(* Logix 5000 AddOnInstructionDefinition export EH_Liquiphant_FTL43_IOL; software revision 38.00 *)

TYPE EH_CommAOI_Data :
STRUCT
   Device_Comm_Error : BOOL;
   CommSuccess : BOOL;
   CommFailed : BOOL;
   CommTimeOut : BOOL;
   StateDone : BOOL;
   NewState : BOOL;
   OldState : SINT;
   PortSize : SINT;
   DevicePort : SINT;
   MaxState : SINT;
   State : SINT;
   VendorID : INT;
   DeviceID : DINT;
   CyclicData : INT[16];
   AcyclicData : DINT[8];
   ReplayIndex : INT;
   AOI_Diagnostic : DINT;
   ConnectionStatus : DINT;
   OutputData : INT[16];
END_STRUCT
END_TYPE

ADD_ON_INSTRUCTION EH_Liquiphant_FTL43_IOL   (* revision 1.2, vendor Endress+Hauser *)
// Liquiphant FTL 43  Rev 1 IO-Link
// Revision note:
// 1.2 Added HeartbeatVerification
// 1.1 Changed the Datatype from Unsigned to Signed
// Add Disconnect check
VAR_IN_OUT
   DataToSend : INT[10]; {required}
   CommAOIBusy : DINT; {required}
   ActiveComPort : DINT; {required}
   DeviceAOISendRequest : DINT; {required}
   CommError : INT; {required}
   DeviceData : EH_CommAOI_Data; {required}
END_VAR
VAR_INPUT
   iSetSimulation : BOOL; {visible}
   iSimulationVariable : INT; {visible}
   iSetSensorFrequency : REAL; {visible}
   iReadStrengthFork : BOOL; {visible}
   iStart_HeartbeatVerification : BOOL; {visible}
END_VAR
VAR_OUTPUT
   qVendor_ID : DINT; {access Read Only, visible}
   qDevice_ID : DINT; {access Read Only, visible}
   qSensorFrequency : REAL; {access None, visible}
   qExtendedDeviceStatus : INT; {access Read Only, visible}
   qSSC1_1 : BOOL; {access Read Only, visible}
   qSSC1_2 : BOOL; {access Read Only, visible}
   qSignalStrengthOfFork : REAL; {access Read Only, visible}
   qVerificationID : DINT; {visible}
   qPassed : BOOL; {access None, visible}
   qFailed : BOOL; {access None, visible}
   qAOI_Diagnostic : DINT; {access Read Only, visible}
END_VAR
VAR_IN_OUT
   qAOI_Diagnostic_String : STRING; {required}
END_VAR
VAR_OUTPUT
   qActual_Diagnostics_Code : DINT; {access Read Only, visible}
END_VAR
VAR_IN_OUT
   qActual_Diagnostics_String : STRING; {required}
END_VAR
VAR_OUTPUT
   qLast_Diagnostics_Code : DINT; {visible}
END_VAR
VAR_IN_OUT
   qLast_Diagnostics_String : STRING; {required}
END_VAR
VAR_OUTPUT
   qCommError : DINT; {access None}
   qCommunicationBusy : DINT; {access Read Only, visible}
   qDeviceConnectionError : BOOL; {access Read Only, visible}
   qFoamIndex : REAL; {access Read Only}
   qFoamDetected : BOOL; {access Read Only}
   qBuildupIndex : REAL; {access Read Only}
   qBuildupDetected : BOOL; {access Read Only}
END_VAR
VAR
   Temp_DINT : DINT; {access None}
   CMD_Index : INT; {access None}
   CMD_Subindex : INT; {access None}
   CMD_ByteLength : INT; {access None}
   oldCondStatus : INT; {access None}
   oldSetSimulation : SINT; {access None}
   SetSimulation : SINT; {access None}
   oldSetUnit : SINT; {access None}
   oldReadStrengthFork : SINT; {access None}
   Trigger : BOOL; {access None}
   CMD_Rd : BOOL; {access None}
   CMD_Wr : BOOL; {access None}
   SimulationDINT : DINT; {access None}
   AOI_Prio : BOOL; {access None}
   StateMin : DINT; {access None}
   firstTimeDone : BOOL; {access None}
   CondStatusChanged : BOOL; {access None}
   Calc_ExtendedDeviceStatus : DINT; {access None}
   Totalizer1_DINT : DINT; {access None}
   SimActive : BOOL; {access None}
   CondStatusActive : BOOL; {access None}
   ActiveAOI : BOOL; {access None}
   Skip : BOOL; {access None}
   SimChanged : BOOL; {access None}
   ReadStrengthFork : SINT; {access None}
   oldStart_HeartbeatVerification : SINT; {access None}
   Start_HeartbeatVerification : SINT; {access None}
   UnitActive : BOOL; {access None}
   UnitChanged : BOOL; {access None}
   DeviceID : DINT; {access None}
   Calc_SensorFrequ : DINT; {access None}
   FALSE : BOOL; {access None}
   TRUE : BOOL := 1; {access None}
   temp_string1 : STRING; {access None}
   temp_string2 : STRING; {access None}
   qFoamIndexDINT : DINT; {access None}
   qFoamDetectedDINT : DINT; {access None}
   qBuildupIndexDINT : DINT; {access None}
   qBuildupDetectedDINT : DINT; {access None}
   qSignalStrengthOfFork_DINT : DINT; {access None}
   ReadStrengthForkChanged : BOOL; {access None}
   ReadStrengthForkActive : BOOL; {access None}
   HeartbeatVerificationActive : BOOL; {access None}
   HeartbeatVerificationChanged : BOOL; {access None}
END_VAR

ROUTINE Logic   (* structured text *)
// Picomag Communication via AL1323
   // =======================================================================
   // Endress+Hauser Digital Solutions
   // ©Copyright (2024) All Rights Reserved
   // =======================================================================
   // Name:                EH_Liquiphant_FTL43_IOL
   // Version:             1.2
   // Datum:               11.2025
   // Library:             01.01.00
   // Engineering:         Studio5000 V38.00.00
   // Author:              EH
   // =======================================================================
   
   qAOI_Diagnostic := DeviceData.AOI_Diagnostic;
   qCommunicationBusy := CommAOIBusy;
   DeviceID := 9559809;
   StateMin := 0;
   DeviceData.MaxState := 98;
   
   if DeviceData.DevicePort = 0 or DeviceData.DeviceID <> DeviceID or DeviceData.ConnectionStatus <> 1 then
   
   	qVendor_ID := DeviceData.VendorID;
   	qDevice_ID := DeviceData.DeviceID;
   	qSensorFrequency	:= 0;
   	qExtendedDeviceStatus	:= 0;
   	qSSC1_1	:= FALSE;
   	qSSC1_2	:= FALSE;
   	qActual_Diagnostics_Code	:= 0;
   	qLast_Diagnostics_Code	:= 0;
   	qLast_Diagnostics_String	:= '';
   	qSignalStrengthOfFork := 0;
   	qPassed := FALSE;
   	qFailed := FALSE;
   	oldCondStatus := 0;
   	CondStatusChanged := FALSE;
   
   	if DeviceData.DevicePort = 0 then
   
   		qActual_Diagnostics_String	:= 'Device Port is Zero';
   		DeviceData.AOI_Diagnostic.1 := TRUE;
   
   	elsif DeviceData.ConnectionStatus <> 1 then
   
   		qActual_Diagnostics_String	:= 'No Device connected';
   		qDeviceConnectionError := TRUE;
   
   	elsif DeviceData.DeviceID <> DeviceID then
   
   		qActual_Diagnostics_String	:= 'Wrong DeviceID';
   		DeviceData.AOI_Diagnostic.2 := TRUE;
   
   	end_if;
   
   else
   
   	if qActual_Diagnostics_Code = 0  then
   
   		qActual_Diagnostics_String	:= '--------';
   
   	end_if;
   
   	if qLast_Diagnostics_Code = 0 then
   
   		qLast_Diagnostics_String	:= '--------';
   
   	end_if;
   
   	DeviceData.AOI_Diagnostic.1 := FALSE;
   	qDeviceConnectionError := FALSE;
   	DeviceData.AOI_Diagnostic.2  := FALSE;
   
   end_if;
   
   // Case device disconnected during communication to avoid blocking the communication
   if (DeviceData.AOI_Diagnostic.0 or qDeviceConnectionError or DeviceData.AOI_Diagnostic.2) and ActiveAOI and ActiveComPort = DeviceData.DevicePort and CommAOIBusy = 1 then
   
   	DeviceData.State := 0;
   	CommAOIBusy := 0;
   	DeviceAOISendRequest.[DeviceData.DevicePort] := 0;
   	ActiveComPort := 0;
   	ActiveAOI := 0;
   	DataToSend[0] := 0;
   	DataToSend[1] := 0;
   	DataToSend[2] := 0;
   	DataToSend[3] := 0;
   	DataToSend[4] := 0;
   	DataToSend[5] := 0;
   	DataToSend[6] := 0;
   	DataToSend[7] := 0;
   	DataToSend[8] := 0;
   	DataToSend[9] := 0;
   	DeviceData.StateDone := FALSE;
   	DeviceData.NewState := FALSE;
   	DeviceData.OldState := 0;
   	ActiveAOI := FALSE;
   
   end_if;
   
   if not DeviceData.AOI_Diagnostic.0
   
   	and not qDeviceConnectionError
   	and not DeviceData.AOI_Diagnostic.2
   	and DeviceData.DevicePort > 0 then
   
   	//*********************************
   	//Vendor ID
   	//*********************************
   
   		qVendor_ID := DeviceData.VendorID;
   
   	//*********************************
   	//Device ID
   	//*********************************
   
   		qDevice_ID := DeviceData.DeviceID;
   
   	//*********************************
   	// FTL43
   	//*********************************
   
   		Calc_SensorFrequ			:= 0;
   		Calc_ExtendedDeviceStatus	:= 2;
   
   	//*********************************
   	//Process Data Level Linearized
   	//*********************************
   
   		Temp_DINT	 := DeviceData.CyclicData[Calc_SensorFrequ+1];
   		Temp_DINT.8	 := DeviceData.CyclicData[Calc_SensorFrequ+1].8;
   		Temp_DINT.9  := DeviceData.CyclicData[Calc_SensorFrequ+1].9;
   		Temp_DINT.10 := DeviceData.CyclicData[Calc_SensorFrequ+1].10;
   		Temp_DINT.11 := DeviceData.CyclicData[Calc_SensorFrequ+1].11;
   		Temp_DINT.12 := DeviceData.CyclicData[Calc_SensorFrequ+1].12;
   		Temp_DINT.13 := DeviceData.CyclicData[Calc_SensorFrequ+1].13;
   		Temp_DINT.14 := DeviceData.CyclicData[Calc_SensorFrequ+1].14;
   		Temp_DINT.15 := DeviceData.CyclicData[Calc_SensorFrequ+1].15;
   		Temp_DINT.16 := DeviceData.CyclicData[Calc_SensorFrequ].0;
   		Temp_DINT.17 := DeviceData.CyclicData[Calc_SensorFrequ].1;
   		Temp_DINT.18 := DeviceData.CyclicData[Calc_SensorFrequ].2;
   		Temp_DINT.19 := DeviceData.CyclicData[Calc_SensorFrequ].3;
   		Temp_DINT.20 := DeviceData.CyclicData[Calc_SensorFrequ].4;
   		Temp_DINT.21 := DeviceData.CyclicData[Calc_SensorFrequ].5;
   		Temp_DINT.22 := DeviceData.CyclicData[Calc_SensorFrequ].6;
   		Temp_DINT.23 := DeviceData.CyclicData[Calc_SensorFrequ].7;
   		Temp_DINT.24 := DeviceData.CyclicData[Calc_SensorFrequ].8;
   		Temp_DINT.25 := DeviceData.CyclicData[Calc_SensorFrequ].9;
   		Temp_DINT.26 := DeviceData.CyclicData[Calc_SensorFrequ].10;
   		Temp_DINT.27 := DeviceData.CyclicData[Calc_SensorFrequ].11;
   		Temp_DINT.28 := DeviceData.CyclicData[Calc_SensorFrequ].12;
   		Temp_DINT.29 := DeviceData.CyclicData[Calc_SensorFrequ].13;
   		Temp_DINT.30 := DeviceData.CyclicData[Calc_SensorFrequ].14;
   		Temp_DINT.31 := DeviceData.CyclicData[Calc_SensorFrequ].15;
   
   		COP(Temp_DINT,qSensorFrequency,1);
   
   	//*********************************
   	// Extended device Status
   	//*********************************
   
   		qExtendedDeviceStatus.0 := DeviceData.CyclicData[Calc_ExtendedDeviceStatus].8;
   		qExtendedDeviceStatus.1 := DeviceData.CyclicData[Calc_ExtendedDeviceStatus].9;
   		qExtendedDeviceStatus.2 := DeviceData.CyclicData[Calc_ExtendedDeviceStatus].10;
   		qExtendedDeviceStatus.3 := DeviceData.CyclicData[Calc_ExtendedDeviceStatus].11;
   		qExtendedDeviceStatus.4 := DeviceData.CyclicData[Calc_ExtendedDeviceStatus].12;
   		qExtendedDeviceStatus.5 := DeviceData.CyclicData[Calc_ExtendedDeviceStatus].13;
   		qExtendedDeviceStatus.6 := DeviceData.CyclicData[Calc_ExtendedDeviceStatus].14;
   		qExtendedDeviceStatus.7 := DeviceData.CyclicData[Calc_ExtendedDeviceStatus].15;
   
   	//*********************************
   	// Process Parameter SSC
   	//*********************************
   
   		qSSC1_1 := DeviceData.CyclicData[Calc_ExtendedDeviceStatus].0;
   		qSSC1_2 := DeviceData.CyclicData[Calc_ExtendedDeviceStatus].1;
   
   	//*********************************
   	// Checking for Changed Status
   	//*********************************
   
   		SetSimulation.0 := iSetSimulation;
   		ReadStrengthFork.0 := iReadStrengthFork;
   		Start_HeartbeatVerification.0 := iStart_HeartbeatVerification;
   
   	if oldCondStatus <> qExtendedDeviceStatus and not CondStatusChanged then
   
   		CondStatusChanged := TRUE;
   		oldCondStatus := qExtendedDeviceStatus;
   
   	end_if;
   
   	if oldSetSimulation <> SetSimulation and not SimChanged then
   
   		if oldSetSimulation < SetSimulation then
   
   			SimChanged := TRUE;
   
   		end_if;
   
   		oldSetSimulation := SetSimulation;
   
   	end_if;
   
   	if oldReadStrengthFork <> ReadStrengthFork and not ReadStrengthForkChanged then
   
   		if oldReadStrengthFork < ReadStrengthFork then
   
   			ReadStrengthForkChanged := TRUE;
   
   		end_if;
   
   		oldReadStrengthFork := ReadStrengthFork;
   
   	end_if;
   
   	if oldStart_HeartbeatVerification <> Start_HeartbeatVerification and not HeartbeatVerificationChanged then
   
   		if oldStart_HeartbeatVerification < Start_HeartbeatVerification then
   
   			HeartbeatVerificationChanged := TRUE;
   
   		end_if;
   
   		oldStart_HeartbeatVerification := Start_HeartbeatVerification;
   
   	end_if;
   
   	if CondStatusChanged
   	and not ActiveAOI
   	and not CondStatusActive
   	and not Skip then
   
   		DeviceAOISendRequest.[DeviceData.DevicePort] := TRUE;
   		CondStatusActive := TRUE;
   		Skip := TRUE;
   
   	elsif SimChanged
   		and not ActiveAOI
   		and not SimActive
   		and not Skip then
   
   		DeviceAOISendRequest.[DeviceData.DevicePort] := TRUE;
   		SimActive := TRUE;
   		Skip := TRUE;
   
   	elsif ReadStrengthForkChanged
   		and not ActiveAOI
   		and not ReadStrengthForkActive
   		and not Skip then
   
   		DeviceAOISendRequest.[DeviceData.DevicePort] := TRUE;
   		ReadStrengthForkActive := TRUE;
   		Skip := TRUE;
   
   	elsif HeartbeatVerificationChanged
   		and not ActiveAOI
   		and not HeartbeatVerificationActive
   		and not Skip then
   
   		DeviceAOISendRequest.[DeviceData.DevicePort] := TRUE;
   		HeartbeatVerificationActive := TRUE;
   		Skip := TRUE;
   
   	end_if;
   
   	if ActiveComPort = DeviceData.DevicePort then
   
   		AOI_Prio := TRUE;
   
   	else
   
   		AOI_Prio := FALSE;
   
   	end_if;
   
   	if (SimActive or ReadStrengthForkActive  or HeartbeatVerificationActive or CondStatusActive) and CommAOIBusy = 1  and DeviceData.State = 0 and AOI_Prio and not ActiveAOI then
   
   		ActiveAOI := TRUE;
   		Skip := FALSE;
   
   	end_if;
   
   	qCommunicationBusy := CommAOIBusy;
   	qAOI_Diagnostic :=DeviceData.AOI_Diagnostic;
   
   	//*********************************
   	// States for Execution
   	//*********************************
   
   	if ActiveAOI or DeviceData.State = DeviceData.MaxState then
   
   	case DeviceData.State of
   
   		//*********************************
   		0: // Idle
   		//*********************************
   
   			// Initializing
   			Trigger := 0;
   			CMD_Index := 0;
   			CMD_Subindex := 0;
   			CMD_Wr := FALSE;
   			CMD_Rd := FALSE;
   		    CMD_ByteLength := 0;
   
   			if DeviceData.DevicePort = ActiveComPort then
   					DeviceData.CommSuccess := FALSE;
   					DeviceData.CommTimeOut := FALSE;
   					DeviceData.NewState := TRUE;
   					DeviceData.StateDone := FALSE;
   				end_if;
   
   			// Wait for trigger
   			if SimActive then
   
   				DeviceData.AOI_Diagnostic := 0;
   				DeviceData.State := 1;
   
   			elsif ReadStrengthForkActive then
   
   				DeviceData.AOI_Diagnostic := 0;
   				DeviceData.State := 12;
   
   			elsif HeartbeatVerificationActive then
   
   				DeviceData.AOI_Diagnostic := 0;
   				DeviceData.State := 80;
   
   			elsif CondStatusChanged then
   
   				DeviceData.State := 90;
   
   			end_if;
   
   	//*********************************
   	1: // Set Simulation Variable
   	//*********************************
   
   			CMD_Index := 1332;
   			CMD_Subindex := 0;
   			CMD_Wr := TRUE;								// Only Read or Write can be active = 1
   			CMD_Rd := FALSE;
   			CMD_ByteLength := 2;
   			DataToSend[6]:= 0;
   			DataToSend[7]:= 0;
   
   			if iSimulationVariable > 0 then
   
   				DataToSend[6].8 := iSimulationVariable.0;
   				DataToSend[6].9 := iSimulationVariable.1;
   				DataToSend[6].10 := iSimulationVariable.2;
   				DataToSend[6].11 := iSimulationVariable.3;
   				DataToSend[6].12 := iSimulationVariable.4;
   				DataToSend[6].13 := iSimulationVariable.5;
   				DataToSend[6].14 := iSimulationVariable.6;
   				DataToSend[6].15 := iSimulationVariable.7;
   
   			else
   				DataToSend[6] := 0;
   				DataToSend[7] := 0;
   			end_if;
   
   			Trigger := TRUE;
   
   			if DeviceData.NewState then
   				DeviceData.StateDone := TRUE;
   			end_if;
   
   			if  DeviceData.CommSuccess and DeviceData.ReplayIndex = CMD_Index then
   
   				Trigger := FALSE;
   				DeviceData.OldState := DeviceData.State;
   				DeviceData.State := DeviceData.State + 1;
   				DeviceData.CommSuccess := FALSE;
   				DeviceData.AcyclicData[0] := 0;
   				DeviceData.NewState := TRUE;
   
   				elsif DeviceData.CommTimeOut then
   
   					temp_string1 := 'Error in step ';
   					Temp_DINT := DeviceData.State;
   					DTOS(Temp_DINT, temp_string2);
   					CONCAT(temp_string1, temp_string2, qAOI_Diagnostic_String);
   
   					DeviceData.OldState := DeviceData.State;
   					DeviceData.State := DeviceData.MaxState;
   					DeviceData.CommTimeOut := FALSE;
   					DeviceData.AcyclicData[0] := 0;
   					DeviceData.NewState := TRUE;
   
   			end_if;
   
   
   		//*********************************
   		2: // Set Simulation Value
   		//*********************************
   
   			CMD_Index := 8738;
   			CMD_Subindex := 0;
   			CMD_Wr := TRUE;								// Only Read or Write can be active = 1
   			CMD_Rd := FALSE;
   			CMD_ByteLength := 4;
   			DataToSend[6]:= 0;
   			DataToSend[7]:= 0;
   
   		 	COP(iSetSensorFrequency,SimulationDINT,1);		// Copy the Bits from the Real in a DINT
   
   			DataToSend[6].0 :=  SimulationDINT.24;
   			DataToSend[6].1 :=  SimulationDINT.25;
   			DataToSend[6].2 :=  SimulationDINT.26;
   			DataToSend[6].3 :=  SimulationDINT.27;
   			DataToSend[6].4 :=  SimulationDINT.28;
   			DataToSend[6].5 :=  SimulationDINT.29;
   			DataToSend[6].6 :=  SimulationDINT.30;
   			DataToSend[6].7 :=  SimulationDINT.31;
   			DataToSend[6].8 :=  SimulationDINT.16;
   			DataToSend[6].9 :=  SimulationDINT.17;
   			DataToSend[6].10 := SimulationDINT.18;
   			DataToSend[6].11 := SimulationDINT.19;
   			DataToSend[6].12 := SimulationDINT.20;
   			DataToSend[6].13 := SimulationDINT.21;
   			DataToSend[6].14 := SimulationDINT.22;
   			DataToSend[6].15 := SimulationDINT.23;
   			DataToSend[7].0  := SimulationDINT.8;
   			DataToSend[7].1  := SimulationDINT.9;
   			DataToSend[7].2  := SimulationDINT.10;
   			DataToSend[7].3  := SimulationDINT.11;
   			DataToSend[7].4  := SimulationDINT.12;
   			DataToSend[7].5  := SimulationDINT.13;
   			DataToSend[7].6  := SimulationDINT.14;
   			DataToSend[7].7  := SimulationDINT.15;
   			DataToSend[7].8  := SimulationDINT.0;
   			DataToSend[7].9  := SimulationDINT.1;
   			DataToSend[7].10 := SimulationDINT.2;
   			DataToSend[7].11 := SimulationDINT.3;
   			DataToSend[7].12 := SimulationDINT.4;
   			DataToSend[7].13 := SimulationDINT.5;
   			DataToSend[7].14 := SimulationDINT.6;
   			DataToSend[7].15 := SimulationDINT.7;
   
   			Trigger := TRUE;
   
   			if DeviceData.NewState then
   				DeviceData.StateDone := TRUE;
   			end_if;
   
   			if  DeviceData.CommSuccess and DeviceData.ReplayIndex = CMD_Index then
   
   				Trigger := FALSE;
   				DeviceData.OldState := DeviceData.State;
   				DeviceData.State := DeviceData.MaxState;
   				DeviceData.CommSuccess := FALSE;
   				DeviceData.AcyclicData[0] := 0;
   				DeviceData.NewState := TRUE;
   
   		 	elsif DeviceData.CommTimeOut then
   
   				temp_string1 := 'Error in step ';
   				Temp_DINT := DeviceData.State;
   				DTOS(Temp_DINT, temp_string2);
   				CONCAT(temp_string1, temp_string2, qAOI_Diagnostic_String);
   
   				DeviceData.OldState := DeviceData.State;
   				DeviceData.State := DeviceData.MaxState;
   				DeviceData.CommTimeOut := FALSE;
   				DeviceData.AcyclicData[0] := 0;
   				DeviceData.NewState := TRUE;
   
   			end_if;
   
   
   		//*********************************
   		12: // Read Signal Strength of Fork
   		//*********************************
   
   			CMD_Index := 4174;
   			CMD_Subindex := 0;
   			CMD_Wr := FALSE;
   			CMD_Rd := TRUE;
   			CMD_ByteLength := 4;
   			Trigger := TRUE;
   
   			if DeviceData.NewState then
   				DeviceData.StateDone := TRUE;
   			end_if;
   
   			if  DeviceData.CommSuccess and DeviceData.ReplayIndex = CMD_Index then
   
   				qSignalStrengthOfFork_DINT	:= DeviceData.AcyclicData[0];
   	 			COP(qSignalStrengthOfFork_DINT, qSignalStrengthOfFork,1);		// Copy the Bits from the Real in a DINT
   
   				Trigger := FALSE;
   				DeviceData.OldState := DeviceData.State;
   				DeviceData.State := DeviceData.MaxState;
   				DeviceData.CommSuccess := FALSE;
   				DeviceData.AcyclicData[0] := 0;
   				DeviceData.NewState := TRUE;
   
   
   			 elsif DeviceData.CommTimeOut then
   
   				temp_string1 := 'Error in step ';
   				Temp_DINT := DeviceData.State;
   				DTOS(Temp_DINT, temp_string2);
   				CONCAT(temp_string1, temp_string2, qAOI_Diagnostic_String);
   
   				DeviceData.OldState := DeviceData.State;
   				DeviceData.State := DeviceData.MaxState;
   				DeviceData.CommTimeOut := FALSE;
   				DeviceData.AcyclicData[0] := 0;
   				DeviceData.NewState := TRUE;
   
   			end_if;
   
   		//*********************************
   		80: // Check Heartbeat Verification activation
   		//*********************************
   			CMD_Index := 12342;
   			CMD_Subindex := 0;
   			CMD_Wr := FALSE;
   			CMD_Rd := TRUE;
   			CMD_ByteLength := 1;
   			Trigger := TRUE;
   			DataToSend[6]:= 0;
   			DataToSend[7]:= 0;
   
   			if DeviceData.NewState then
   
   				DeviceData.StateDone := TRUE;
   
   			end_if;
   
   			if  DeviceData.CommSuccess and DeviceData.ReplayIndex = CMD_Index then
   
   				if DeviceData.AcyclicData[0] = 1 then
   
   					DeviceData.State := DeviceData.State + 1;
   
   				else
   					qAOI_Diagnostic_String := 'Step 80: Software Option not activated ';
   
   					DeviceData.OldState := DeviceData.State;
   					DeviceData.State := DeviceData.MaxState;
   
   				end_if;
   
   				Trigger := FALSE;
   				DeviceData.CommSuccess := FALSE;
   				DeviceData.AcyclicData[0] := 0;
   				DeviceData.NewState := TRUE;
   
   			 elsif DeviceData.CommTimeOut then
   
   				temp_string1 := 'Error in step ';
   				Temp_DINT := DeviceData.State;
   				DTOS(Temp_DINT, temp_string2);
   				CONCAT(temp_string1, temp_string2, qAOI_Diagnostic_String);
   
   				DeviceData.OldState := DeviceData.State;
   				DeviceData.State := DeviceData.MaxState;
   				DeviceData.CommTimeOut := FALSE;
   				DeviceData.AcyclicData[0] := 0;
   				DeviceData.NewState := TRUE;
   
   			end_if;
   
   		//*********************************
   		81: // Check if Verifivation is ongoing
   		//*********************************
   			CMD_Index := 12323;
   			CMD_Subindex := 0;
   			CMD_Wr := FALSE;
   			CMD_Rd := TRUE;
   			CMD_ByteLength := 2;
   			Trigger := TRUE;
   
   			if DeviceData.NewState then
   
   				DeviceData.StateDone := TRUE;
   
   			end_if;
   
   			if  DeviceData.CommSuccess and DeviceData.ReplayIndex = CMD_Index then
   
   				if DeviceData.AcyclicData[0] <> 8 then
   
   					DeviceData.State := DeviceData.State + 1;
   
   				else
   					qAOI_Diagnostic_String := 'Step 81: Heartbeat Verification already in progress ';
   					DeviceData.OldState := DeviceData.State;
   					DeviceData.State := DeviceData.MaxState;
   					DeviceData.CommTimeOut := FALSE;
   
   				end_if;
   
   				Trigger := FALSE;
   				DeviceData.CommSuccess := FALSE;
   				DeviceData.AcyclicData[0] := 0;
   				DeviceData.NewState := TRUE;
   
   			 elsif DeviceData.CommTimeOut then
   
   				temp_string1 := 'Error in step ';
   				Temp_DINT := DeviceData.State;
   				DTOS(Temp_DINT, temp_string2);
   				CONCAT(temp_string1, temp_string2, qAOI_Diagnostic_String);
   
   				DeviceData.OldState := DeviceData.State;
   				DeviceData.State := DeviceData.MaxState;
   				DeviceData.CommTimeOut := FALSE;
   				DeviceData.AcyclicData[0] := 0;
   				DeviceData.NewState := TRUE;
   
   			end_if;
   
   		//*********************************
   		82: // Start Verification
   		//*********************************
   			CMD_Index := 12325;
   			CMD_Subindex := 0;
   			CMD_Wr := TRUE;
   			CMD_Rd := FALSE;
   			CMD_ByteLength := 2;
   			Trigger := TRUE;
   			DataToSend[6] := 0;
   			DataToSend[7] := 0;
   
   			DataToSend[6].8 := TRUE;
   
   			if DeviceData.NewState then
   
   				DeviceData.StateDone := TRUE;
   
   			end_if;
   
   		if DeviceData.CommSuccess and DeviceData.ReplayIndex = CMD_Index then
   
   		    Trigger := FALSE;
   		    DeviceData.CommSuccess := FALSE;
   		    DeviceData.State := DeviceData.State + 3;
   			DeviceData.AcyclicData[0] := 0;
   			DeviceData.NewState := TRUE;
   
   		elsif DeviceData.CommTimeOut then
   
   		    temp_string1 := 'Error in step ';
   		    Temp_DINT := DeviceData.State;
   		    DTOS(Temp_DINT, temp_string2);
   		    CONCAT(temp_string1, temp_string2, qAOI_Diagnostic_String);
   
   		    DeviceData.OldState := DeviceData.State;
   		    DeviceData.State := DeviceData.MaxState;
   		    DeviceData.CommTimeOut := FALSE;
   			DeviceData.AcyclicData[0] := 0;
   			DeviceData.NewState := TRUE;
   
   		end_if;
   
   
   		//*********************************
   		83: // Intermediate state
   		//*********************************
   			CMD_Index := 36;
   			CMD_Subindex := 0;
   			CMD_Wr := FALSE;
   			CMD_Rd := TRUE;
   			CMD_ByteLength := 1;
   			Trigger := TRUE;
   
   			if DeviceData.NewState then
   
   				DeviceData.StateDone := TRUE;
   
   			end_if;
   
   			if DeviceData.CommSuccess and DeviceData.ReplayIndex = CMD_Index then
   
   			    DeviceData.State := DeviceData.State + 2;
   			    Trigger := FALSE;
   			    DeviceData.CommSuccess := FALSE;
   				DeviceData.AcyclicData[0] := 0;
   				DeviceData.NewState := TRUE;
   
   			elsif DeviceData.CommTimeOut then
   
   			    temp_string1 := 'Error in step ';
   			    Temp_DINT := DeviceData.State;
   			    DTOS(Temp_DINT, temp_string2);
   			    CONCAT(temp_string1, temp_string2, qAOI_Diagnostic_String);
   
   			    DeviceData.OldState := DeviceData.State;
   			    DeviceData.State := DeviceData.MaxState;
   			    DeviceData.CommTimeOut := FALSE;
   				DeviceData.AcyclicData[0] := 0;
   				DeviceData.NewState := TRUE;
   
   			end_if;
   
   		//*********************************
   		84: // Read progress
   		//*********************************
   
   		//*********************************
   		85: // Read status
   		//*********************************
   			CMD_Index := 12323;
   			CMD_Subindex := 0;
   			CMD_Wr := FALSE;
   			CMD_Rd := TRUE;
   			CMD_ByteLength := 2;
   			Trigger := TRUE;
   
   			if DeviceData.NewState then
   
   				DeviceData.StateDone := TRUE;
   
   			end_if;
   
   			if DeviceData.CommSuccess and DeviceData.ReplayIndex = CMD_Index then
   
   			    if DeviceData.AcyclicData[0] = 10 then
   
   			        DeviceData.State := DeviceData.State + 1;
   
   			    elsif DeviceData.AcyclicData[0] = 8 then
   
   					DeviceData.State := DeviceData.State - 2;
   
   			    else
   			        qAOI_Diagnostic_String := 'Step 85: Heartbeat Verification not done';
   			        DeviceData.OldState := DeviceData.State;
   			        DeviceData.State := DeviceData.MaxState;
   			        DeviceData.CommTimeOut := FALSE;
   
   			    end_if;
   
   			    Trigger := FALSE;
   			    DeviceData.CommSuccess := FALSE;
   				DeviceData.AcyclicData[0] := 0;
   				DeviceData.NewState := TRUE;
   
   			elsif DeviceData.CommTimeOut then
   
   			    temp_string1 := 'Error in step ';
   			    Temp_DINT := DeviceData.State;
   			    DTOS(Temp_DINT, temp_string2);
   			    CONCAT(temp_string1, temp_string2, qAOI_Diagnostic_String);
   
   			    DeviceData.OldState := DeviceData.State;
   			    DeviceData.State := DeviceData.MaxState;
   			    DeviceData.CommTimeOut := FALSE;
   				DeviceData.AcyclicData[0] := 0;
   				DeviceData.NewState := TRUE;
   
   			end_if;
   
   		//*********************************
   		86: // Read overall result
   		//*********************************
   			CMD_Index := 1396;
   			CMD_Subindex := 0;
   			CMD_Wr := FALSE;
   			CMD_Rd := TRUE;
   			CMD_ByteLength := 2;
   			Trigger := TRUE;
   
   			if DeviceData.NewState then
   
   				DeviceData.StateDone := TRUE;
   
   			end_if;
   
   			if  DeviceData.CommSuccess and DeviceData.ReplayIndex = CMD_Index then
   
   				if DeviceData.AcyclicData[0] = 1 then
   
   					qPassed := TRUE;
   					qFailed := FALSE;
   
   				else
   
   					qPassed := FALSE;
   					qFailed := TRUE;
   
   				end_if;
   
   				Trigger := FALSE;
   				DeviceData.CommSuccess := FALSE;
   				DeviceData.State := DeviceData.State + 1;
   				DeviceData.AcyclicData[0] := 0;
   				DeviceData.NewState := TRUE;
   
   			 elsif DeviceData.CommTimeOut then
   
   				temp_string1 := 'Error in step ';
   				Temp_DINT := DeviceData.State;
   				DTOS(Temp_DINT, temp_string2);
   				CONCAT(temp_string1, temp_string2, qAOI_Diagnostic_String);
   
   				DeviceData.CommTimeOut := FALSE;
   				DeviceData.OldState := DeviceData.State;
   				DeviceData.State := DeviceData.MaxState;
   				DeviceData.AcyclicData[0] := 0;
   				DeviceData.NewState := TRUE;
   
   			end_if;
   
   		//*********************************
   		87: // Read Verification ID
   		//*********************************
   			CMD_Index := 12321;
   			CMD_Subindex := 0;
   			CMD_Wr := FALSE;
   			CMD_Rd := TRUE;
   			CMD_ByteLength := 2;
   			Trigger := TRUE;
   
   			if DeviceData.NewState then
   
   				DeviceData.StateDone := TRUE;
   
   			end_if;
   
   			if  DeviceData.CommSuccess and DeviceData.ReplayIndex = CMD_Index then
   
   				qVerificationID.0	:= DeviceData.AcyclicData[0].0;
   				qVerificationID.1	:= DeviceData.AcyclicData[0].1;
   				qVerificationID.2	:= DeviceData.AcyclicData[0].2;
   				qVerificationID.3	:= DeviceData.AcyclicData[0].3;
   				qVerificationID.4	:= DeviceData.AcyclicData[0].4;
   				qVerificationID.5	:= DeviceData.AcyclicData[0].5;
   				qVerificationID.6	:= DeviceData.AcyclicData[0].6;
   				qVerificationID.7	:= DeviceData.AcyclicData[0].7;
   				qVerificationID.8	:= DeviceData.AcyclicData[0].8;
   				qVerificationID.9	:= DeviceData.AcyclicData[0].9;
   				qVerificationID.10	:= DeviceData.AcyclicData[0].10;
   				qVerificationID.11	:= DeviceData.AcyclicData[0].11;
   				qVerificationID.12	:= DeviceData.AcyclicData[0].12;
   				qVerificationID.13	:= DeviceData.AcyclicData[0].13;
   				qVerificationID.14	:= DeviceData.AcyclicData[0].14;
   				qVerificationID.15	:= DeviceData.AcyclicData[0].15;
   
   				Trigger := FALSE;
   				DeviceData.CommSuccess := FALSE;
   				DeviceData.OldState := DeviceData.State;
   				DeviceData.State := DeviceData.MaxState;
   				DeviceData.NewState := TRUE;
   
   			 elsif DeviceData.CommTimeOut then
   
   				temp_string1 := 'Error in step ';
   				Temp_DINT := DeviceData.State;
   				DTOS(Temp_DINT, temp_string2);
   				CONCAT(temp_string1, temp_string2, qAOI_Diagnostic_String);
   
   				DeviceData.CommTimeOut := FALSE;
   				DeviceData.OldState := DeviceData.State;
   				DeviceData.State := DeviceData.MaxState;
   				DeviceData.NewState := TRUE;
   
   			end_if;
   
   		//*********************************
   		90: // Actual Diagnostic
   		//*********************************
   
   			CMD_Index := 297;
   			CMD_Subindex := 0;
   			CMD_Wr := FALSE;
   			CMD_Rd := TRUE;
   			CMD_ByteLength := 4;
   			Trigger := TRUE;
   
   			if DeviceData.NewState then
   
   				DeviceData.StateDone := TRUE;
   
   			end_if;
   
   			if  DeviceData.CommSuccess and DeviceData.ReplayIndex = CMD_Index then
   
   				qActual_Diagnostics_Code	:= DeviceData.AcyclicData[0];
   
   				case qActual_Diagnostics_Code of
   
     					0:
   			            qActual_Diagnostics_String := '--------';
   			        16777245:
   			            qActual_Diagnostics_String := 'F081 Sensor initialization faulty';
   			        16777250:
   			            qActual_Diagnostics_String := 'F062 Sensor connection faulty';
   			        16777259:
   			            qActual_Diagnostics_String := 'F801 Supply voltage too low';
   			        16777283:
   			            qActual_Diagnostics_String := 'F803 Loop current faulty';
   			        16777312:
   			            qActual_Diagnostics_String := 'F437 Configuration incompatible';
   			        16777314:
   			            qActual_Diagnostics_String := 'F282 Data storage inconsistent';
   			        16777319:
   			            qActual_Diagnostics_String := 'F242 Firmware incompatible';
   			        16777323:
   			            qActual_Diagnostics_String := 'F252 Module incompatible';
   			        16777336:
   			            qActual_Diagnostics_String := 'F270 Main electronics defective';
   			        16777337:
   			            qActual_Diagnostics_String := 'F272 Main electronics faulty';
   			        16777340:
   			            qActual_Diagnostics_String := 'F270 Main electronics defective';
   			        16777341:
   			            qActual_Diagnostics_String := 'F272 Main electronics faulty';
   			        16777343:
   			            qActual_Diagnostics_String := 'F270 Main electronics defective';
   			        16777344:
   			            qActual_Diagnostics_String := 'F270 Main electronics defective';
   			        16777348:
   			            qActual_Diagnostics_String := 'F270 Main electronics defective';
   			        16777351:
   			            qActual_Diagnostics_String := 'F825 Electronics temperature out of range';
   			        16777355:
   			            qActual_Diagnostics_String := 'F410 Data transfer failed';
   			        16777374:
   			            qActual_Diagnostics_String := 'F283 Memory content inconsistent';
   			        16777375:
   			            qActual_Diagnostics_String := 'F270 Main electronics defective';
   			        16777387:
   			            qActual_Diagnostics_String := 'F270 Main electronics defective';
   			        16777389:
   			            qActual_Diagnostics_String := 'F805 Loop current faulty';
   			        16777441:
   			            qActual_Diagnostics_String := 'F283 Memory content inconsistent';
   			        16777445:
   			            qActual_Diagnostics_String := 'F273 Main electronics defective';
   			        16777446:
   			            qActual_Diagnostics_String := 'F388 Electronics and HistoROM defective';
   			        16777816:
   			            qActual_Diagnostics_String := 'F272 Main electronics faulty';
   			        16778157:
   			            qActual_Diagnostics_String := 'F201 Electronics faulty';
   			        16778194:
   			            qActual_Diagnostics_String := 'F826 Sensor temperature out of range';
   			        16778253:
   			            qActual_Diagnostics_String := 'F062 Sensor connection faulty';
   			        16778254:
   			            qActual_Diagnostics_String := 'F062 Sensor connection faulty';
   			        16778255:
   			            qActual_Diagnostics_String := 'F062 Sensor connection faulty';
   			        16778256:
   			            qActual_Diagnostics_String := 'F062 Sensor connection faulty';
   			        16778279:
   			            qActual_Diagnostics_String := 'F806 Current-loop values deviated';
   			        16778295:
   			            qActual_Diagnostics_String := 'F272 Main electronics faulty';
   			        16778436:
   			            qActual_Diagnostics_String := 'F901 Process alert frequency too high';
   			        16778437:
   			            qActual_Diagnostics_String := 'F900 Process alert frequency too low';
   			        16778445:
   			            qActual_Diagnostics_String := 'F842 Process limit';
   			        16778446:
   			            qActual_Diagnostics_String := 'F007 Sensor defective';
   			        16778447:
   			            qActual_Diagnostics_String := 'F049 Sensor corroded';
   			        16778448:
   			            qActual_Diagnostics_String := 'F042 Sensor corroded';
   			        16778449:
   			            qActual_Diagnostics_String := 'F061 Sensor electronics faulty';
   			        16778457:
   			            qActual_Diagnostics_String := 'F061 Sensor electronics faulty';
   			        16778459:
   			            qActual_Diagnostics_String := 'F061 Sensor electronics faulty';
   			        16778490:
   			            qActual_Diagnostics_String := 'F419 Power cycle required';
   			        16778684:
   			            qActual_Diagnostics_String := 'F004 Sensor defective';
   			        16778685:
   			            qActual_Diagnostics_String := 'F004 Sensor defective';
   			        16778686:
   			            qActual_Diagnostics_String := 'F004 Sensor defective';
   			        16778687:
   			            qActual_Diagnostics_String := 'F004 Sensor defective';
   			        16778688:
   			            qActual_Diagnostics_String := 'F004 Sensor defective';
   			        16778689:
   			            qActual_Diagnostics_String := 'F004 Sensor defective';
   			        16778690:
   			            qActual_Diagnostics_String := 'F004 Sensor defective';
   			        16778691:
   			            qActual_Diagnostics_String := 'F004 Sensor defective';
   			        16778692:
   			            qActual_Diagnostics_String := 'F004 Sensor defective';
   			        16778693:
   			            qActual_Diagnostics_String := 'F004 Sensor defective';
   			        16778694:
   			            qActual_Diagnostics_String := 'F004 Sensor defective';
   			        16778695:
   			            qActual_Diagnostics_String := 'F004 Sensor defective';
   			        16778696:
   			            qActual_Diagnostics_String := 'F004 Sensor defective';
   			        16778697:
   			            qActual_Diagnostics_String := 'F004 Sensor defective';
   			        16778698:
   			            qActual_Diagnostics_String := 'F004 Sensor defective';
   			        16778699:
   			            qActual_Diagnostics_String := 'F004 Sensor defective';
   			        16778700:
   			            qActual_Diagnostics_String := 'F004 Sensor defective';
   			        16778701:
   			            qActual_Diagnostics_String := 'F004 Sensor defective';
   			        16778702:
   			            qActual_Diagnostics_String := 'F004 Sensor defective';
   			        16778703:
   			            qActual_Diagnostics_String := 'F004 Sensor defective';
   			        25165853:
   			            qActual_Diagnostics_String := 'F081 Sensor initialization faulty';
   			        25165858:
   			            qActual_Diagnostics_String := 'F062 Sensor connection faulty';
   			        25165867:
   			            qActual_Diagnostics_String := 'F801 Supply voltage too low';
   			        25165891:
   			            qActual_Diagnostics_String := 'F803 Loop current faulty';
   			        25165920:
   			            qActual_Diagnostics_String := 'F437 Configuration incompatible';
   			        25165922:
   			            qActual_Diagnostics_String := 'F282 Data storage inconsistent';
   			        25165927:
   			            qActual_Diagnostics_String := 'F242 Firmware incompatible';
   			        25165931:
   			            qActual_Diagnostics_String := 'F252 Module incompatible';
   			        25165944:
   			            qActual_Diagnostics_String := 'F270 Main electronics defective';
   			        25165945:
   			            qActual_Diagnostics_String := 'F272 Main electronics faulty';
   			        25165948:
   			            qActual_Diagnostics_String := 'F270 Main electronics defective';
   			        25165949:
   			            qActual_Diagnostics_String := 'F272 Main electronics faulty';
   			        25165951:
   			            qActual_Diagnostics_String := 'F270 Main electronics defective';
   			        25165952:
   			            qActual_Diagnostics_String := 'F270 Main electronics defective';
   			        25165956:
   			            qActual_Diagnostics_String := 'F270 Main electronics defective';
   			        25165959:
   			            qActual_Diagnostics_String := 'F825 Electronics temperature out of range';
   			        25165963:
   			            qActual_Diagnostics_String := 'F410 Data transfer failed';
   			        25165982:
   			            qActual_Diagnostics_String := 'F283 Memory content inconsistent';
   			        25165983:
   			            qActual_Diagnostics_String := 'F270 Main electronics defective';
   			        25165995:
   			            qActual_Diagnostics_String := 'F270 Main electronics defective';
   			        25165997:
   			            qActual_Diagnostics_String := 'F805 Loop current faulty';
   			        25166049:
   			            qActual_Diagnostics_String := 'F283 Memory content inconsistent';
   			        25166053:
   			            qActual_Diagnostics_String := 'F273 Main electronics defective';
   			        25166054:
   			            qActual_Diagnostics_String := 'F388 Electronics and HistoROM defective';
   			        25166424:
   			            qActual_Diagnostics_String := 'F272 Main electronics faulty';
   			        25166765:
   			            qActual_Diagnostics_String := 'F201 Electronics faulty';
   			        25166802:
   			            qActual_Diagnostics_String := 'F826 Sensor temperature out of range';
   			        25166861:
   			            qActual_Diagnostics_String := 'F062 Sensor connection faulty';
   			        25166862:
   			            qActual_Diagnostics_String := 'F062 Sensor connection faulty';
   			        25166863:
   			            qActual_Diagnostics_String := 'F062 Sensor connection faulty';
   			        25166864:
   			            qActual_Diagnostics_String := 'F062 Sensor connection faulty';
   			        25166887:
   			            qActual_Diagnostics_String := 'F806 Current-loop values deviated';
   			        25166903:
   			            qActual_Diagnostics_String := 'F272 Main electronics faulty';
   			        25167044:
   			            qActual_Diagnostics_String := 'F901 Process alert frequency too high';
   			        25167045:
   			            qActual_Diagnostics_String := 'F900 Process alert frequency too low';
   			        25167053:
   			            qActual_Diagnostics_String := 'F842 Process limit';
   			        25167054:
   			            qActual_Diagnostics_String := 'F007 Sensor defective';
   			        25167055:
   			            qActual_Diagnostics_String := 'F049 Sensor corroded';
   			        25167056:
   			            qActual_Diagnostics_String := 'F042 Sensor corroded';
   			        25167057:
   			            qActual_Diagnostics_String := 'F061 Sensor electronics faulty';
   			        25167065:
   			            qActual_Diagnostics_String := 'F061 Sensor electronics faulty';
   			        25167067:
   			            qActual_Diagnostics_String := 'F061 Sensor electronics faulty';
   			        25167098:
   			            qActual_Diagnostics_String := 'F419 Power cycle required';
   			        25167292:
   			            qActual_Diagnostics_String := 'F004 Sensor defective';
   			        25167293:
   			            qActual_Diagnostics_String := 'F004 Sensor defective';
   			        25167294:
   			            qActual_Diagnostics_String := 'F004 Sensor defective';
   			        25167295:
   			            qActual_Diagnostics_String := 'F004 Sensor defective';
   			        25167296:
   			            qActual_Diagnostics_String := 'F004 Sensor defective';
   			        25167297:
   			            qActual_Diagnostics_String := 'F004 Sensor defective';
   			        25167298:
   			            qActual_Diagnostics_String := 'F004 Sensor defective';
   			        25167299:
   			            qActual_Diagnostics_String := 'F004 Sensor defective';
   			        25167300:
   			            qActual_Diagnostics_String := 'F004 Sensor defective';
   			        25167301:
   			            qActual_Diagnostics_String := 'F004 Sensor defective';
   			        25167302:
   			            qActual_Diagnostics_String := 'F004 Sensor defective';
   			        25167303:
   			            qActual_Diagnostics_String := 'F004 Sensor defective';
   			        25167304:
   			            qActual_Diagnostics_String := 'F004 Sensor defective';
   			        25167305:
   			            qActual_Diagnostics_String := 'F004 Sensor defective';
   			        25167306:
   			            qActual_Diagnostics_String := 'F004 Sensor defective';
   			        25167307:
   			            qActual_Diagnostics_String := 'F004 Sensor defective';
   			        25167308:
   			            qActual_Diagnostics_String := 'F004 Sensor defective';
   			        25167309:
   			            qActual_Diagnostics_String := 'F004 Sensor defective';
   			        25167310:
   			            qActual_Diagnostics_String := 'F004 Sensor defective';
   			        25167311:
   			            qActual_Diagnostics_String := 'F004 Sensor defective';
   			        33554445:
   			            qActual_Diagnostics_String := 'C485 Process variable simulation active';
   			        33554446:
   			            qActual_Diagnostics_String := 'C491 Current output simulation active';
   			        33554567:
   			            qActual_Diagnostics_String := 'C825 Electronics temperature out of range';
   			        33554575:
   			            qActual_Diagnostics_String := 'C494 Switch output simulation active';
   			        33554576:
   			            qActual_Diagnostics_String := 'C484 Failure mode simulation active';
   			        33554948:
   			            qActual_Diagnostics_String := 'C412 Processing download';
   			        33555410:
   			            qActual_Diagnostics_String := 'C826 Sensor temperature out of range';
   			        33555459:
   			            qActual_Diagnostics_String := 'C490 Output simulation';
   			        33555495:
   			            qActual_Diagnostics_String := 'C806 Current-loop values deviated';
   			        33555652:
   			            qActual_Diagnostics_String := 'C901 Process alert frequency too high';
   			        33555653:
   			            qActual_Diagnostics_String := 'C900 Process alert frequency too low';
   			        33555654:
   			            qActual_Diagnostics_String := 'C485 Process variable simulation active';
   			        33555660:
   			            qActual_Diagnostics_String := 'C485 Process variable simulation active';
   			        33555663:
   			            qActual_Diagnostics_String := 'C049 Sensor corroded';
   			        33555674:
   			            qActual_Diagnostics_String := 'C485 Process variable simulation active';
   			        41943053:
   			            qActual_Diagnostics_String := 'C485 Process variable simulation active';
   			        41943054:
   			            qActual_Diagnostics_String := 'C491 Current output simulation active';
   			        41943175:
   			            qActual_Diagnostics_String := 'C825 Electronics temperature out of range';
   			        41943183:
   			            qActual_Diagnostics_String := 'C494 Switch output simulation active';
   			        41943184:
   			            qActual_Diagnostics_String := 'C484 Failure mode simulation active';
   			        41943556:
   			            qActual_Diagnostics_String := 'C412 Processing download';
   			        41944018:
   			            qActual_Diagnostics_String := 'C826 Sensor temperature out of range';
   			        41944067:
   			            qActual_Diagnostics_String := 'C490 Output simulation';
   			        41944103:
   			            qActual_Diagnostics_String := 'C806 Current-loop values deviated';
   			        41944260:
   			            qActual_Diagnostics_String := 'C901 Process alert frequency too high';
   			        41944261:
   			            qActual_Diagnostics_String := 'C900 Process alert frequency too low';
   			        41944262:
   			            qActual_Diagnostics_String := 'C485 Process variable simulation active';
   			        41944268:
   			            qActual_Diagnostics_String := 'C485 Process variable simulation active';
   			        41944271:
   			            qActual_Diagnostics_String := 'C049 Sensor corroded';
   			        41944282:
   			            qActual_Diagnostics_String := 'C485 Process variable simulation active';
   			        67108868:
   			            qActual_Diagnostics_String := 'M431 Trim required';
   			        67108970:
   			            qActual_Diagnostics_String := 'M438 Dataset different';
   			        67108999:
   			            qActual_Diagnostics_String := 'M825 Electronics temperature out of range';
   			        67109090:
   			            qActual_Diagnostics_String := 'M287 Memory content inconsistent';
   			        67109839:
   			            qActual_Diagnostics_String := 'M538 Configuration Sensor Unit invalid';
   			        67109842:
   			            qActual_Diagnostics_String := 'M826 Sensor temperature out of range';
   			        67109896:
   			            qActual_Diagnostics_String := 'M807 No Baseline due to insuf. volt. at 20 mA';
   			        67109927:
   			            qActual_Diagnostics_String := 'M806 Current-loop values deviated';
   			        67109944:
   			            qActual_Diagnostics_String := 'M287 Memory content inconsistent';
   			        67110084:
   			            qActual_Diagnostics_String := 'M901 Process alert frequency too high';
   			        67110085:
   			            qActual_Diagnostics_String := 'M900 Process alert frequency too low';
   			        67110095:
   			            qActual_Diagnostics_String := 'M049 Sensor corroded';
   			        75497476:
   			            qActual_Diagnostics_String := 'M431 Trim required';
   			        75497578:
   			            qActual_Diagnostics_String := 'M438 Dataset different';
   			        75497607:
   			            qActual_Diagnostics_String := 'M825 Electronics temperature out of range';
   			        75497698:
   			            qActual_Diagnostics_String := 'M287 Memory content inconsistent';
   			        75498447:
   			            qActual_Diagnostics_String := 'M538 Configuration Sensor Unit invalid';
   			        75498450:
   			            qActual_Diagnostics_String := 'M826 Sensor temperature out of range';
   			        75498504:
   			            qActual_Diagnostics_String := 'M807 No Baseline due to insuf. volt. at 20 mA';
   			        75498535:
   			            qActual_Diagnostics_String := 'M806 Current-loop values deviated';
   			        75498552:
   			            qActual_Diagnostics_String := 'M287 Memory content inconsistent';
   			        75498692:
   			            qActual_Diagnostics_String := 'M901 Process alert frequency too high';
   			        75498693:
   			            qActual_Diagnostics_String := 'M900 Process alert frequency too low';
   			        75498703:
   			            qActual_Diagnostics_String := 'M049 Sensor corroded';
   			        134217772:
   			            qActual_Diagnostics_String := 'S802 Supply voltage too high';
   			        134217863:
   			            qActual_Diagnostics_String := 'S825 Electronics temperature out of range';
   			        134217881:
   			            qActual_Diagnostics_String := 'S441 Current output saturated';
   			        134218194:
   			            qActual_Diagnostics_String := 'S946 Vibration detected';
   			        134218639:
   			            qActual_Diagnostics_String := 'S804 Switch output overloaded';
   			        134218706:
   			            qActual_Diagnostics_String := 'S826 Sensor temperature out of range';
   			        134218791:
   			            qActual_Diagnostics_String := 'S806 Current-loop values deviated';
   			        134218948:
   			            qActual_Diagnostics_String := 'S901 Process alert frequency too high';
   			        134218949:
   			            qActual_Diagnostics_String := 'S900 Process alert frequency too low';
   			        134218959:
   			            qActual_Diagnostics_String := 'S049 Sensor corroded';
   			        142606380:
   			            qActual_Diagnostics_String := 'S802 Supply voltage too high';
   			        142606471:
   			            qActual_Diagnostics_String := 'S825 Electronics temperature out of range';
   			        142606489:
   			            qActual_Diagnostics_String := 'S441 Current output saturated';
   			        142606802:
   			            qActual_Diagnostics_String := 'S946 Vibration detected';
   			        142607247:
   			            qActual_Diagnostics_String := 'S804 Switch output overloaded';
   			        142607314:
   			            qActual_Diagnostics_String := 'S826 Sensor temperature out of range';
   			        142607399:
   			            qActual_Diagnostics_String := 'S806 Current-loop values deviated';
   			        142607556:
   			            qActual_Diagnostics_String := 'S901 Process alert frequency too high';
   			        142607557:
   			            qActual_Diagnostics_String := 'S900 Process alert frequency too low';
   			        142607567:
   			            qActual_Diagnostics_String := 'S049 Sensor corroded';
   			        536871047:
   			            qActual_Diagnostics_String := '825 Electronics temperature out of range';
   			        536871262:
   			            qActual_Diagnostics_String := '495 Diagnostic event simulation active';
   			        536871890:
   			            qActual_Diagnostics_String := '826 Sensor temperature out of range';
   			        536871975:
   			            qActual_Diagnostics_String := '806 Current-loop values deviated';
   			        536872132:
   			            qActual_Diagnostics_String := '901 Process alert frequency too high';
   			        536872133:
   			            qActual_Diagnostics_String := '900 Process alert frequency too low';
   			        536872143:
   			            qActual_Diagnostics_String := '049 Sensor corroded';
   			        545259655:
   			            qActual_Diagnostics_String := '825 Electronics temperature out of range';
   			        545259870:
   			            qActual_Diagnostics_String := '495 Diagnostic event simulation active';
   			        545260498:
   			            qActual_Diagnostics_String := '826 Sensor temperature out of range';
   			        545260583:
   			            qActual_Diagnostics_String := '806 Current-loop values deviated';
   			        545260740:
   			            qActual_Diagnostics_String := '901 Process alert frequency too high';
   			        545260741:
   			            qActual_Diagnostics_String := '900 Process alert frequency too low';
   			        545260751:
   			            qActual_Diagnostics_String := '049 Sensor corroded';
   					else
   						qActual_Diagnostics_String := 'Error Code unknown';
   
   				end_case;
   
   				Trigger := FALSE;
   				DeviceData.OldState := DeviceData.State;
   		        DeviceData.State := DeviceData.State+1;
   				DeviceData.CommSuccess := FALSE;
   				DeviceData.AcyclicData[0] := 0;
   				DeviceData.NewState := TRUE;
   
   			 elsif DeviceData.CommTimeOut then
   
   				temp_string1 := 'Error in step ';
   				Temp_DINT := DeviceData.State;
   				DTOS(Temp_DINT, temp_string2);
   				CONCAT(temp_string1, temp_string2, qAOI_Diagnostic_String);
   
   				DeviceData.OldState := DeviceData.State;
   				DeviceData.State := DeviceData.State + 1;
   				DeviceData.CommTimeOut := FALSE;
   				DeviceData.AcyclicData[0] := 0;
   				DeviceData.NewState := TRUE;
   
   		    end_if;
   
   		//*********************************
   	    91: // Last Diagnostic
   	    //*********************************
   
   		    CMD_Index := 298;
   			CMD_Subindex := 0;
   		    CMD_Wr := FALSE;
   			CMD_Rd := TRUE;
   			CMD_ByteLength := 4;
   			Trigger := TRUE;
   
   			if DeviceData.NewState then
   
   				DeviceData.StateDone := TRUE;
   
   			end_if;
   
   			if  DeviceData.CommSuccess and DeviceData.ReplayIndex = CMD_Index then
   
   				qLast_Diagnostics_Code	:= DeviceData.AcyclicData[0];
   
   				case qLast_Diagnostics_Code of
   					0:
   			            qLast_Diagnostics_String := '--------';
   			        16777245:
   			            qLast_Diagnostics_String := 'F081 Sensor initialization faulty';
   			        16777250:
   			            qLast_Diagnostics_String := 'F062 Sensor connection faulty';
   			        16777259:
   			            qLast_Diagnostics_String := 'F801 Supply voltage too low';
   			        16777283:
   			            qLast_Diagnostics_String := 'F803 Loop current faulty';
   			        16777312:
   			            qLast_Diagnostics_String := 'F437 Configuration incompatible';
   			        16777314:
   			            qLast_Diagnostics_String := 'F282 Data storage inconsistent';
   			        16777319:
   			            qLast_Diagnostics_String := 'F242 Firmware incompatible';
   			        16777323:
   			            qLast_Diagnostics_String := 'F252 Module incompatible';
   			        16777336:
   			            qLast_Diagnostics_String := 'F270 Main electronics defective';
   			        16777337:
   			            qLast_Diagnostics_String := 'F272 Main electronics faulty';
   			        16777340:
   			            qLast_Diagnostics_String := 'F270 Main electronics defective';
   			        16777341:
   			            qLast_Diagnostics_String := 'F272 Main electronics faulty';
   			        16777343:
   			            qLast_Diagnostics_String := 'F270 Main electronics defective';
   			        16777344:
   			            qLast_Diagnostics_String := 'F270 Main electronics defective';
   			        16777348:
   			            qLast_Diagnostics_String := 'F270 Main electronics defective';
   			        16777351:
   			            qLast_Diagnostics_String := 'F825 Electronics temperature out of range';
   			        16777355:
   			            qLast_Diagnostics_String := 'F410 Data transfer failed';
   			        16777374:
   			            qLast_Diagnostics_String := 'F283 Memory content inconsistent';
   			        16777375:
   			            qLast_Diagnostics_String := 'F270 Main electronics defective';
   			        16777387:
   			            qLast_Diagnostics_String := 'F270 Main electronics defective';
   			        16777389:
   			            qLast_Diagnostics_String := 'F805 Loop current faulty';
   			        16777441:
   			            qLast_Diagnostics_String := 'F283 Memory content inconsistent';
   			        16777445:
   			            qLast_Diagnostics_String := 'F273 Main electronics defective';
   			        16777446:
   			            qLast_Diagnostics_String := 'F388 Electronics and HistoROM defective';
   			        16777816:
   			            qLast_Diagnostics_String := 'F272 Main electronics faulty';
   			        16778157:
   			            qLast_Diagnostics_String := 'F201 Electronics faulty';
   			        16778194:
   			            qLast_Diagnostics_String := 'F826 Sensor temperature out of range';
   			        16778253:
   			            qLast_Diagnostics_String := 'F062 Sensor connection faulty';
   			        16778254:
   			            qLast_Diagnostics_String := 'F062 Sensor connection faulty';
   			        16778255:
   			            qLast_Diagnostics_String := 'F062 Sensor connection faulty';
   			        16778256:
   			            qLast_Diagnostics_String := 'F062 Sensor connection faulty';
   			        16778279:
   			            qLast_Diagnostics_String := 'F806 Current-loop values deviated';
   			        16778295:
   			            qLast_Diagnostics_String := 'F272 Main electronics faulty';
   			        16778436:
   			            qLast_Diagnostics_String := 'F901 Process alert frequency too high';
   			        16778437:
   			            qLast_Diagnostics_String := 'F900 Process alert frequency too low';
   			        16778445:
   			            qLast_Diagnostics_String := 'F842 Process limit';
   			        16778446:
   			            qLast_Diagnostics_String := 'F007 Sensor defective';
   			        16778447:
   			            qLast_Diagnostics_String := 'F049 Sensor corroded';
   			        16778448:
   			            qLast_Diagnostics_String := 'F042 Sensor corroded';
   			        16778449:
   			            qLast_Diagnostics_String := 'F061 Sensor electronics faulty';
   			        16778457:
   			            qLast_Diagnostics_String := 'F061 Sensor electronics faulty';
   			        16778459:
   			            qLast_Diagnostics_String := 'F061 Sensor electronics faulty';
   			        16778490:
   			            qLast_Diagnostics_String := 'F419 Power cycle required';
   			        16778684:
   			            qLast_Diagnostics_String := 'F004 Sensor defective';
   			        16778685:
   			            qLast_Diagnostics_String := 'F004 Sensor defective';
   			        16778686:
   			            qLast_Diagnostics_String := 'F004 Sensor defective';
   			        16778687:
   			            qLast_Diagnostics_String := 'F004 Sensor defective';
   			        16778688:
   			            qLast_Diagnostics_String := 'F004 Sensor defective';
   			        16778689:
   			            qLast_Diagnostics_String := 'F004 Sensor defective';
   			        16778690:
   			            qLast_Diagnostics_String := 'F004 Sensor defective';
   			        16778691:
   			            qLast_Diagnostics_String := 'F004 Sensor defective';
   			        16778692:
   			            qLast_Diagnostics_String := 'F004 Sensor defective';
   			        16778693:
   			            qLast_Diagnostics_String := 'F004 Sensor defective';
   			        16778694:
   			            qLast_Diagnostics_String := 'F004 Sensor defective';
   			        16778695:
   			            qLast_Diagnostics_String := 'F004 Sensor defective';
   			        16778696:
   			            qLast_Diagnostics_String := 'F004 Sensor defective';
   			        16778697:
   			            qLast_Diagnostics_String := 'F004 Sensor defective';
   			        16778698:
   			            qLast_Diagnostics_String := 'F004 Sensor defective';
   			        16778699:
   			            qLast_Diagnostics_String := 'F004 Sensor defective';
   			        16778700:
   			            qLast_Diagnostics_String := 'F004 Sensor defective';
   			        16778701:
   			            qLast_Diagnostics_String := 'F004 Sensor defective';
   			        16778702:
   			            qLast_Diagnostics_String := 'F004 Sensor defective';
   			        16778703:
   			            qLast_Diagnostics_String := 'F004 Sensor defective';
   			        25165853:
   			            qLast_Diagnostics_String := 'F081 Sensor initialization faulty';
   			        25165858:
   			            qLast_Diagnostics_String := 'F062 Sensor connection faulty';
   			        25165867:
   			            qLast_Diagnostics_String := 'F801 Supply voltage too low';
   			        25165891:
   			            qLast_Diagnostics_String := 'F803 Loop current faulty';
   			        25165920:
   			            qLast_Diagnostics_String := 'F437 Configuration incompatible';
   			        25165922:
   			            qLast_Diagnostics_String := 'F282 Data storage inconsistent';
   			        25165927:
   			            qLast_Diagnostics_String := 'F242 Firmware incompatible';
   			        25165931:
   			            qLast_Diagnostics_String := 'F252 Module incompatible';
   			        25165944:
   			            qLast_Diagnostics_String := 'F270 Main electronics defective';
   			        25165945:
   			            qLast_Diagnostics_String := 'F272 Main electronics faulty';
   			        25165948:
   			            qLast_Diagnostics_String := 'F270 Main electronics defective';
   			        25165949:
   			            qLast_Diagnostics_String := 'F272 Main electronics faulty';
   			        25165951:
   			            qLast_Diagnostics_String := 'F270 Main electronics defective';
   			        25165952:
   			            qLast_Diagnostics_String := 'F270 Main electronics defective';
   			        25165956:
   			            qLast_Diagnostics_String := 'F270 Main electronics defective';
   			        25165959:
   			            qLast_Diagnostics_String := 'F825 Electronics temperature out of range';
   			        25165963:
   			            qLast_Diagnostics_String := 'F410 Data transfer failed';
   			        25165982:
   			            qLast_Diagnostics_String := 'F283 Memory content inconsistent';
   			        25165983:
   			            qLast_Diagnostics_String := 'F270 Main electronics defective';
   			        25165995:
   			            qLast_Diagnostics_String := 'F270 Main electronics defective';
   			        25165997:
   			            qLast_Diagnostics_String := 'F805 Loop current faulty';
   			        25166049:
   			            qLast_Diagnostics_String := 'F283 Memory content inconsistent';
   			        25166053:
   			            qLast_Diagnostics_String := 'F273 Main electronics defective';
   			        25166054:
   			            qLast_Diagnostics_String := 'F388 Electronics and HistoROM defective';
   			        25166424:
   			            qLast_Diagnostics_String := 'F272 Main electronics faulty';
   			        25166765:
   			            qLast_Diagnostics_String := 'F201 Electronics faulty';
   			        25166802:
   			            qLast_Diagnostics_String := 'F826 Sensor temperature out of range';
   			        25166861:
   			            qLast_Diagnostics_String := 'F062 Sensor connection faulty';
   			        25166862:
   			            qLast_Diagnostics_String := 'F062 Sensor connection faulty';
   			        25166863:
   			            qLast_Diagnostics_String := 'F062 Sensor connection faulty';
   			        25166864:
   			            qLast_Diagnostics_String := 'F062 Sensor connection faulty';
   			        25166887:
   			            qLast_Diagnostics_String := 'F806 Current-loop values deviated';
   			        25166903:
   			            qLast_Diagnostics_String := 'F272 Main electronics faulty';
   			        25167044:
   			            qLast_Diagnostics_String := 'F901 Process alert frequency too high';
   			        25167045:
   			            qLast_Diagnostics_String := 'F900 Process alert frequency too low';
   			        25167053:
   			            qLast_Diagnostics_String := 'F842 Process limit';
   			        25167054:
   			            qLast_Diagnostics_String := 'F007 Sensor defective';
   			        25167055:
   			            qLast_Diagnostics_String := 'F049 Sensor corroded';
   			        25167056:
   			            qLast_Diagnostics_String := 'F042 Sensor corroded';
   			        25167057:
   			            qLast_Diagnostics_String := 'F061 Sensor electronics faulty';
   			        25167065:
   			            qLast_Diagnostics_String := 'F061 Sensor electronics faulty';
   			        25167067:
   			            qLast_Diagnostics_String := 'F061 Sensor electronics faulty';
   			        25167098:
   			            qLast_Diagnostics_String := 'F419 Power cycle required';
   			        25167292:
   			            qLast_Diagnostics_String := 'F004 Sensor defective';
   			        25167293:
   			            qLast_Diagnostics_String := 'F004 Sensor defective';
   			        25167294:
   			            qLast_Diagnostics_String := 'F004 Sensor defective';
   			        25167295:
   			            qLast_Diagnostics_String := 'F004 Sensor defective';
   			        25167296:
   			            qLast_Diagnostics_String := 'F004 Sensor defective';
   			        25167297:
   			            qLast_Diagnostics_String := 'F004 Sensor defective';
   			        25167298:
   			            qLast_Diagnostics_String := 'F004 Sensor defective';
   			        25167299:
   			            qLast_Diagnostics_String := 'F004 Sensor defective';
   			        25167300:
   			            qLast_Diagnostics_String := 'F004 Sensor defective';
   			        25167301:
   			            qLast_Diagnostics_String := 'F004 Sensor defective';
   			        25167302:
   			            qLast_Diagnostics_String := 'F004 Sensor defective';
   			        25167303:
   			            qLast_Diagnostics_String := 'F004 Sensor defective';
   			        25167304:
   			            qLast_Diagnostics_String := 'F004 Sensor defective';
   			        25167305:
   			            qLast_Diagnostics_String := 'F004 Sensor defective';
   			        25167306:
   			            qLast_Diagnostics_String := 'F004 Sensor defective';
   			        25167307:
   			            qLast_Diagnostics_String := 'F004 Sensor defective';
   			        25167308:
   			            qLast_Diagnostics_String := 'F004 Sensor defective';
   			        25167309:
   			            qLast_Diagnostics_String := 'F004 Sensor defective';
   			        25167310:
   			            qLast_Diagnostics_String := 'F004 Sensor defective';
   			        25167311:
   			            qLast_Diagnostics_String := 'F004 Sensor defective';
   			        33554445:
   			            qLast_Diagnostics_String := 'C485 Process variable simulation active';
   			        33554446:
   			            qLast_Diagnostics_String := 'C491 Current output simulation active';
   			        33554567:
   			            qLast_Diagnostics_String := 'C825 Electronics temperature out of range';
   			        33554575:
   			            qLast_Diagnostics_String := 'C494 Switch output simulation active';
   			        33554576:
   			            qLast_Diagnostics_String := 'C484 Failure mode simulation active';
   			        33554948:
   			            qLast_Diagnostics_String := 'C412 Processing download';
   			        33555410:
   			            qLast_Diagnostics_String := 'C826 Sensor temperature out of range';
   			        33555459:
   			            qLast_Diagnostics_String := 'C490 Output simulation';
   			        33555495:
   			            qLast_Diagnostics_String := 'C806 Current-loop values deviated';
   			        33555652:
   			            qLast_Diagnostics_String := 'C901 Process alert frequency too high';
   			        33555653:
   			            qLast_Diagnostics_String := 'C900 Process alert frequency too low';
   			        33555654:
   			            qLast_Diagnostics_String := 'C485 Process variable simulation active';
   			        33555660:
   			            qLast_Diagnostics_String := 'C485 Process variable simulation active';
   			        33555663:
   			            qLast_Diagnostics_String := 'C049 Sensor corroded';
   			        33555674:
   			            qLast_Diagnostics_String := 'C485 Process variable simulation active';
   			        41943053:
   			            qLast_Diagnostics_String := 'C485 Process variable simulation active';
   			        41943054:
   			            qLast_Diagnostics_String := 'C491 Current output simulation active';
   			        41943175:
   			            qLast_Diagnostics_String := 'C825 Electronics temperature out of range';
   			        41943183:
   			            qLast_Diagnostics_String := 'C494 Switch output simulation active';
   			        41943184:
   			            qLast_Diagnostics_String := 'C484 Failure mode simulation active';
   			        41943556:
   			            qLast_Diagnostics_String := 'C412 Processing download';
   			        41944018:
   			            qLast_Diagnostics_String := 'C826 Sensor temperature out of range';
   			        41944067:
   			            qLast_Diagnostics_String := 'C490 Output simulation';
   			        41944103:
   			            qLast_Diagnostics_String := 'C806 Current-loop values deviated';
   			        41944260:
   			            qLast_Diagnostics_String := 'C901 Process alert frequency too high';
   			        41944261:
   			            qLast_Diagnostics_String := 'C900 Process alert frequency too low';
   			        41944262:
   			            qLast_Diagnostics_String := 'C485 Process variable simulation active';
   			        41944268:
   			            qLast_Diagnostics_String := 'C485 Process variable simulation active';
   			        41944271:
   			            qLast_Diagnostics_String := 'C049 Sensor corroded';
   			        41944282:
   			            qLast_Diagnostics_String := 'C485 Process variable simulation active';
   			        67108868:
   			            qLast_Diagnostics_String := 'M431 Trim required';
   			        67108970:
   			            qLast_Diagnostics_String := 'M438 Dataset different';
   			        67108999:
   			            qLast_Diagnostics_String := 'M825 Electronics temperature out of range';
   			        67109090:
   			            qLast_Diagnostics_String := 'M287 Memory content inconsistent';
   			        67109839:
   			            qLast_Diagnostics_String := 'M538 Configuration Sensor Unit invalid';
   			        67109842:
   			            qLast_Diagnostics_String := 'M826 Sensor temperature out of range';
   			        67109896:
   			            qLast_Diagnostics_String := 'M807 No Baseline due to insuf. volt. at 20 mA';
   			        67109927:
   			            qLast_Diagnostics_String := 'M806 Current-loop values deviated';
   			        67109944:
   			            qLast_Diagnostics_String := 'M287 Memory content inconsistent';
   			        67110084:
   			            qLast_Diagnostics_String := 'M901 Process alert frequency too high';
   			        67110085:
   			            qLast_Diagnostics_String := 'M900 Process alert frequency too low';
   			        67110095:
   			            qLast_Diagnostics_String := 'M049 Sensor corroded';
   			        75497476:
   			            qLast_Diagnostics_String := 'M431 Trim required';
   			        75497578:
   			            qLast_Diagnostics_String := 'M438 Dataset different';
   			        75497607:
   			            qLast_Diagnostics_String := 'M825 Electronics temperature out of range';
   			        75497698:
   			            qLast_Diagnostics_String := 'M287 Memory content inconsistent';
   			        75498447:
   			            qLast_Diagnostics_String := 'M538 Configuration Sensor Unit invalid';
   			        75498450:
   			            qLast_Diagnostics_String := 'M826 Sensor temperature out of range';
   			        75498504:
   			            qLast_Diagnostics_String := 'M807 No Baseline due to insuf. volt. at 20 mA';
   			        75498535:
   			            qLast_Diagnostics_String := 'M806 Current-loop values deviated';
   			        75498552:
   			            qLast_Diagnostics_String := 'M287 Memory content inconsistent';
   			        75498692:
   			            qLast_Diagnostics_String := 'M901 Process alert frequency too high';
   			        75498693:
   			            qLast_Diagnostics_String := 'M900 Process alert frequency too low';
   			        75498703:
   			            qLast_Diagnostics_String := 'M049 Sensor corroded';
   			        134217772:
   			            qLast_Diagnostics_String := 'S802 Supply voltage too high';
   			        134217863:
   			            qLast_Diagnostics_String := 'S825 Electronics temperature out of range';
   			        134217881:
   			            qLast_Diagnostics_String := 'S441 Current output saturated';
   			        134218194:
   			            qLast_Diagnostics_String := 'S946 Vibration detected';
   			        134218639:
   			            qLast_Diagnostics_String := 'S804 Switch output overloaded';
   			        134218706:
   			            qLast_Diagnostics_String := 'S826 Sensor temperature out of range';
   			        134218791:
   			            qLast_Diagnostics_String := 'S806 Current-loop values deviated';
   			        134218948:
   			            qLast_Diagnostics_String := 'S901 Process alert frequency too high';
   			        134218949:
   			            qLast_Diagnostics_String := 'S900 Process alert frequency too low';
   			        134218959:
   			            qLast_Diagnostics_String := 'S049 Sensor corroded';
   			        142606380:
   			            qLast_Diagnostics_String := 'S802 Supply voltage too high';
   			        142606471:
   			            qLast_Diagnostics_String := 'S825 Electronics temperature out of range';
   			        142606489:
   			            qLast_Diagnostics_String := 'S441 Current output saturated';
   			        142606802:
   			            qLast_Diagnostics_String := 'S946 Vibration detected';
   			        142607247:
   			            qLast_Diagnostics_String := 'S804 Switch output overloaded';
   			        142607314:
   			            qLast_Diagnostics_String := 'S826 Sensor temperature out of range';
   			        142607399:
   			            qLast_Diagnostics_String := 'S806 Current-loop values deviated';
   			        142607556:
   			            qLast_Diagnostics_String := 'S901 Process alert frequency too high';
   			        142607557:
   			            qLast_Diagnostics_String := 'S900 Process alert frequency too low';
   			        142607567:
   			            qLast_Diagnostics_String := 'S049 Sensor corroded';
   			        536871047:
   			            qLast_Diagnostics_String := '825 Electronics temperature out of range';
   			        536871262:
   			            qLast_Diagnostics_String := '495 Diagnostic event simulation active';
   			        536871890:
   			            qLast_Diagnostics_String := '826 Sensor temperature out of range';
   			        536871975:
   			            qLast_Diagnostics_String := '806 Current-loop values deviated';
   			        536872132:
   			            qLast_Diagnostics_String := '901 Process alert frequency too high';
   			        536872133:
   			            qLast_Diagnostics_String := '900 Process alert frequency too low';
   			        536872143:
   			            qLast_Diagnostics_String := '049 Sensor corroded';
   			        545259655:
   			            qLast_Diagnostics_String := '825 Electronics temperature out of range';
   			        545259870:
   			            qLast_Diagnostics_String := '495 Diagnostic event simulation active';
   			        545260498:
   			            qLast_Diagnostics_String := '826 Sensor temperature out of range';
   			        545260583:
   			            qLast_Diagnostics_String := '806 Current-loop values deviated';
   			        545260740:
   			            qLast_Diagnostics_String := '901 Process alert frequency too high';
   			        545260741:
   			            qLast_Diagnostics_String := '900 Process alert frequency too low';
   			        545260751:
   			            qLast_Diagnostics_String := '049 Sensor corroded';
   
   					else
   						qLast_Diagnostics_String := 'Error Code unknown';
   
   				end_case;
   
   				Trigger := FALSE;
   				DeviceData.OldState := DeviceData.State;
   		        DeviceData.State := DeviceData.MaxState;
   				DeviceData.CommSuccess := FALSE;
   				DeviceData.AcyclicData[0] := 0;
   				DeviceData.NewState := TRUE;
   
   			 elsif DeviceData.CommTimeOut then
   
   				temp_string1 := 'Error in step ';
   				Temp_DINT := DeviceData.State;
   				DTOS(Temp_DINT, temp_string2);
   				CONCAT(temp_string1, temp_string2, qAOI_Diagnostic_String);
   
   				DeviceData.OldState := DeviceData.State;
   		        DeviceData.State := DeviceData.MaxState;
   				DeviceData.CommTimeOut := FALSE;
   				DeviceData.AcyclicData[0] := 0;
   				DeviceData.NewState := TRUE;
   
   			end_if;
   
   		//*********************************
   		98: // End Step Trigger Guard
   		//*********************************
   
   				DeviceData.State := 0;
   				CommAOIBusy := 0;
   				DeviceAOISendRequest.[DeviceData.DevicePort] := 0;
   				ActiveComPort := 0;
   				ActiveAOI := 0;
   				DataToSend[0] := 0;
   				DataToSend[1] := 0;
   				DataToSend[2] := 0;
   				DataToSend[3] := 0;
   				DataToSend[4] := 0;
   				DataToSend[5] := 0;
    				DataToSend[6] := 0;
   				DataToSend[7] := 0;
    				DataToSend[8] := 0;
   				DataToSend[9] := 0;
   				DeviceData.StateDone := FALSE;
   				Skip := 0;
   				firstTimeDone := FALSE;
   				DeviceData.NewState := FALSE;
   				DeviceData.OldState := 0;
   				ActiveAOI := FALSE;
   
   				if SimActive then
   
   					SimActive := FALSE;
   					SimChanged := FALSE;
   
   				elsif ReadStrengthForkActive then
   
   					ReadStrengthForkActive := FALSE;
   					ReadStrengthForkChanged := FALSE;
   
   				elsif HeartbeatVerificationActive then
   
   					HeartbeatVerificationActive := FALSE;
   					HeartbeatVerificationChanged := FALSE;
   
   				elsif CondStatusActive then
   
   					CondStatusActive := FALSE;
   					CondStatusChanged := FALSE;
   
   				end_if;
   
   	end_case;
   
   	end_if;
   
   	//*************************
   	// Execution Area
   	//*************************
   	if DeviceData.State > StateMin and DeviceData.State < DeviceData.MaxState then
   
   		DataToSend[2] := DeviceData.DevicePort;
   		DataToSend[3] := CMD_Index;
   		DataToSend[4] := CMD_Subindex;
   		DataToSend[5].0 := CMD_Rd;
   		DataToSend[5].1 := CMD_Wr;
   		DataToSend[5].8 := CMD_ByteLength.0;  // Bits for the Length of the Data
   		DataToSend[5].9 := CMD_ByteLength.1;
   		DataToSend[5].10 := CMD_ByteLength.2;
   		DataToSend[5].11 := CMD_ByteLength.3;
   		DataToSend[5].12 := CMD_ByteLength.4;
   		DataToSend[5].13 := CMD_ByteLength.5;
   		DataToSend[5].14 := CMD_ByteLength.6;
   		DataToSend[5].15 := CMD_ByteLength.7;
   		DataToSend[5].7 := Trigger;
   
   		qCommError := CommError;
   
   	end_if;
   
   end_if;
   
   
END_ROUTINE
END_ADD_ON_INSTRUCTION
